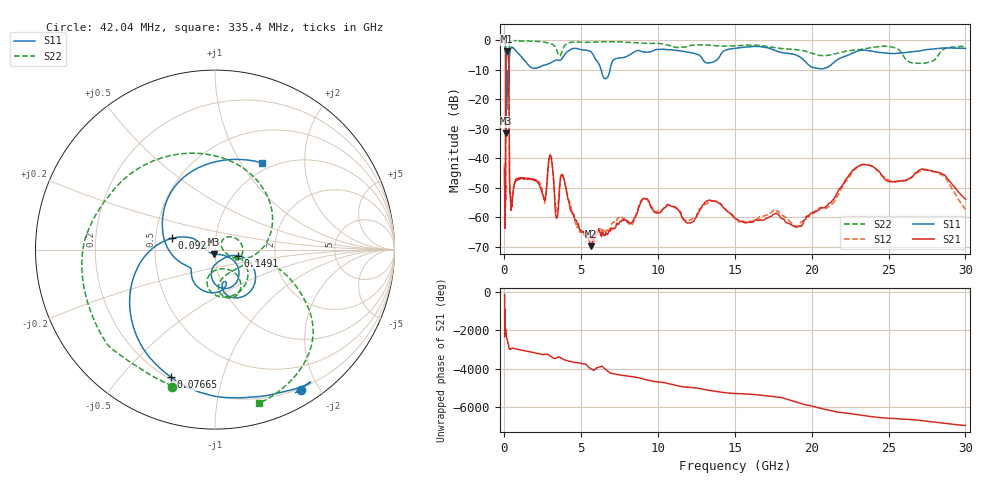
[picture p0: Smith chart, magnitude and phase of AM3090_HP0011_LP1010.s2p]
! Date/Time: Thu, Feb 28, 2019 1:56 PM
! Network Analyzer: Agilent Technologies E8364B Rev: A.07.50.67
! Sweep from 0.010 to 30.000 GHz, 1601 Points, Sweep Type: LOG
! Power Supply: 5.023 V, 0.002 A
# Hz S DB R 50
!freq MagS11 AngS11 MagS21 AngS21 MagS12 AngS12 MagS22 AngS22
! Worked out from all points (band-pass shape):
!   1601 points, 10 MHz to 30 GHz, reference 50 ohm
!   highest |S21| = -3.81 dB at 152.9 MHz (marker M1); lowest = -69.7 dB at 5.64 GHz (marker M2)
!   |S21| within 3 dB of the highest: 103 MHz to 270.7 MHz (167.7 MHz wide, 89.8 % of centre)
!   lowest |S11| = -31.5 dB at 100.9 MHz (marker M3), VSWR 1.05, Z = 49.5 - j2.59 ohm
!   |S11| at or under -10 dB: 91.54 MHz to 298.3 MHz (206.8 MHz wide, 106 % of centre); 6.288 GHz to 6.876 GHz (588 MHz wide, 8.93 % of centre)
!   |S22| runs from -28.1 to -0.2 dB; largest |S21 - S12| = 0.012
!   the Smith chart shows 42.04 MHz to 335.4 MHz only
!   S11 on the Smith chart (normalised r, x): 42.04 MHz: 0.17, -1.78; 76.65 MHz: 0.21, -0.69; 92.7 MHz: 0.61, +0.08; 149.1 MHz: 1.29, -0.09; 335.4 MHz: 0.90, +1.24
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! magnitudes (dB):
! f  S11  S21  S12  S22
! 10 MHz  -0.3  -49.3  -41.8  -0.7
! 38.04 MHz  -0.5  -60.0  -56.6  -1.6
! 42.04 MHz  -0.7  -62.8  -59.9  -1.9
! 76.65 MHz  -2.5  -47.3  -46.2  -4.6
! 92.7 MHz  -12.1  -14.9  -15.0  -11.9
! 100.9 MHz  -31.5  -7.5  -7.5  -27.3
! 116.7 MHz  -13.0  -5.0  -5.0  -17.7
! 144.7 MHz  -21.6  -3.9  -3.8  -18.3
! 149.1 MHz  -17.6  -3.8  -3.8  -17.3
! 152.9 MHz  -15.1  -3.8  -3.8  -16.1
! 274.6 MHz  -15.0  -7.4  -7.4  -16.2
! 335.4 MHz  -5.2  -47.7  -47.7  -1.0
! 550.5 MHz  -2.6  -52.2  -51.8  -0.3
! 2.084 GHz  -9.6  -47.7  -47.4  -0.5
! 3.002 GHz  -7.7  -39.1  -39.1  -1.2
! 3.385 GHz  -6.8  -60.3  -58.0  -3.3
! 3.798 GHz  -5.9  -45.8  -45.9  -3.2
! 5.64 GHz  -4.1  -69.7  -67.3  -0.8
! 7.926 GHz  -5.6  -60.8  -60.9  -0.8
! 19.03 GHz  -5.2  -63.3  -62.9  -3.3
! 23.48 GHz  -3.4  -42.2  -42.0  -2.9
! 30 GHz  -2.8  -53.8  -57.3  -2.2
